{attribute 'no_assign'}
{attribute 'call_after_init'}
FUNCTION_BLOCK FB_IED_IED EXTENDS FB_AcsiCommonIntelligentElectronicDeviceClass
VAR_INPUT
	IEDMUnn: FB_LD_IEDMUnn := (bLinkResult:=THIS^.AddLogicalDeviceToContainer(ipLogicalDevice:=IEDMUnn)); (*Merging unit*)
END_VAR
VAR
END_VAR

END_FUNCTION_BLOCK
